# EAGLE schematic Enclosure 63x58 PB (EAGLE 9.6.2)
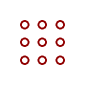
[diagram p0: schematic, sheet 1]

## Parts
U$1  PROTO-20X18  [PROTO-20X18]

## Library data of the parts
U$1 = digitalconcepts:PROTO-20X18: 20 x 18 Prototyping board to fit a 63 x 58 enclosure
